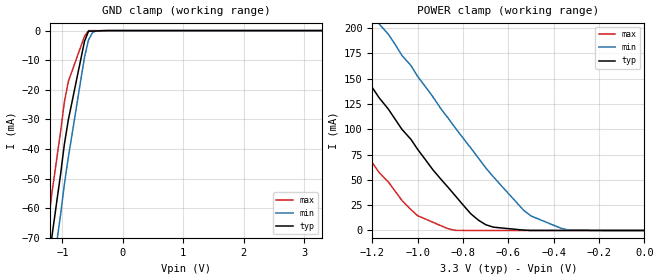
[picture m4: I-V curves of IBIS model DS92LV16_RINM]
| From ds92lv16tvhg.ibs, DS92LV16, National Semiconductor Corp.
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[Model]   DS92LV16_RINM
Model_type Input
Vinh=.1
Vinl=-.1
C_comp   2.922pF   2.922pF   2.922pF
[Temperature Range] 25   85   -40
[Voltage Range]   3.3   3.15   3.45
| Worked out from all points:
|   GND clamp passes 1 mA (typ) near -0.58 V on its own axis
|   POWER clamp passes 1 mA (typ) near -0.56 V on its own axis
[GND Clamp]
|V(groundclamp)   I(typ)   I(min)   I(max)
-3.3V     -416mA     -429mA     -402mA
-1.3V     -89.7mA    -104mA     -74.9mA
-1.23V    -79.3mA    -93mA      -64.5mA
-1.17V    -69.1mA    -82.7mA    -54.4mA
-1.1V     -58.8mA    -72.5mA    -44.3mA
-1.03V    -48.6mA    -62.2mA    -34.2mA
-967mV    -38.4mA    -51.9mA    -24.1mA
-900mV    -30mA      -42.6mA    -17.1mA
-633mV    -3.57mA    -8.92mA    -1.9mA
-567mV    -239uA     -3.14mA    -420nA
-433mV    -133uA     -61.9uA    -233nA
3.3V      21.4pA     6.6nA      19.7pA
[POWER Clamp]
|Vtable   I(typ)   I(min)   I(max)
-3.3V     826mA      900mA      750mA
-1.63V    280mA      354mA      203mA
-1.6V     269mA      344mA      193mA
-1.37V    194mA      268mA      118mA
-1.17V    131mA      204mA      57.1mA
-1.13V    120mA      194mA      48mA
-1V       80mA       152mA      14.5mA
-833mV    33.9mA     101mA      60uA
-700mV    5.68mA     61.9mA     6.68uA
-533mV    372uA      20mA       1.71nA
-366mV    1.1uA      2.03mA     12.8pA
0V        6.66pA     6.59nA     6.3pA
